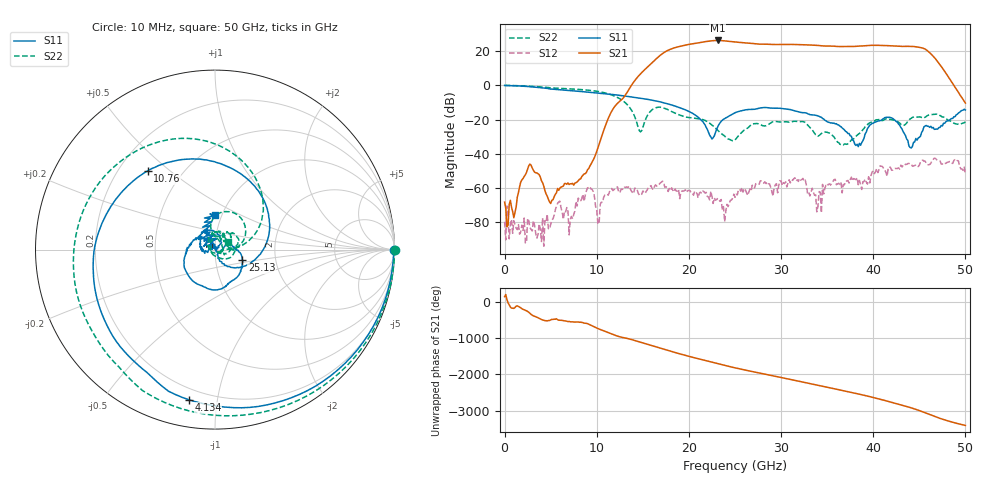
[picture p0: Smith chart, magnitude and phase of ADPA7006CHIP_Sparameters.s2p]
! Analog Devices Inc.
! Device:  ADPA7006CHIP
! Description: GaAs pHEMT MMIC Wide Band Amplifier.
! Frequency:  18.00 -  44.00 GHz
! Package:
! Conditions:	Vdd = 5.0 V
!		Idd = 800 mA
!		Temp = +25 C
! Calibration: Reference at probe tip
! Misc:DB
! Freq(GHz)	S11a(dB)	S11p(deg)	S21a(dB)	S21p(deg)	S12a(dB)	S12p(deg)	S22a(dB)	S22p(deg)
# GHz S  dB  R 50
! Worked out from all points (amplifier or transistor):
!   401 points, 10 MHz to 50 GHz, reference 50 ohm
!   highest |S21| = 26.4 dB at 23.13 GHz (marker M1)
!   |S21| within 3 dB of that: 19.41 GHz to 34.14 GHz (14.73 GHz wide, 55 % of centre)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
!   unconditionally stable (mu >= 1): 139.1 MHz to end of sweep
!   at 8.258 GHz: K = 157716.19, MAG = -48.6 dB, |S12| = -67.6 dB
!   at 25.01 GHz: K = 49.53, MAG = 25.6 dB, |S12| = -65.6 dB
!   at 50 GHz: K = 649.07, MAG = -10.1 dB, |S12| = -52.3 dB
!   S11 on the Smith chart (normalised r, x): 10 MHz: open; 4.134 GHz: 0.14, -0.83; 10.76 GHz: 0.32, +0.42; 25.13 GHz: 1.35, -0.16; 50 GHz: 0.93, +0.37
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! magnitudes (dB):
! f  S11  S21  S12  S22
! 10 MHz  0.0  -68.4  -80.0  0.0
! 1.01 GHz  -0.2  -77.6  -79.3  -0.1
! 2.759 GHz  -0.7  -46.1  -83.4  -0.5
! 4.134 GHz  -1.4  -57.1  -77.7  -0.9
! 5.009 GHz  -2.1  -69.2  -81.4  -1.5
! 8.383 GHz  -3.6  -53.4  -66.5  -2.5
! 9.383 GHz  -4.1  -46.2  -60.7  -3.0
! 10.13 GHz  -4.5  -36.7  -80.9  -3.5
! 10.76 GHz  -4.8  -26.4  -65.6  -4.2
! 14.76 GHz  -7.5  6.8  -64.5  -27.2
! 16.76 GHz  -9.5  17.0  -58.1  -12.7
! 23.13 GHz  -24.4  26.4  -66.1  -26.3
! 23.88 GHz  -19.5  26.1  -79.9  -29.7
! 25.01 GHz  -16.1  25.5  -65.6  -31.9
! 25.13 GHz  -15.7  25.4  -63.8  -31.3
! 31.38 GHz  -14.7  24.0  -54.7  -21.1
! 33.38 GHz  -17.3  23.7  -60.3  -26.1
! 38.38 GHz  -35.9  23.0  -58.2  -28.6
! 41.75 GHz  -18.7  23.3  -47.7  -19.9
! 44.13 GHz  -36.7  22.8  -46.0  -19.3
! 46.38 GHz  -25.0  17.9  -44.1  -17.1
! 50 GHz  -14.4  -10.3  -52.3  -21.3
